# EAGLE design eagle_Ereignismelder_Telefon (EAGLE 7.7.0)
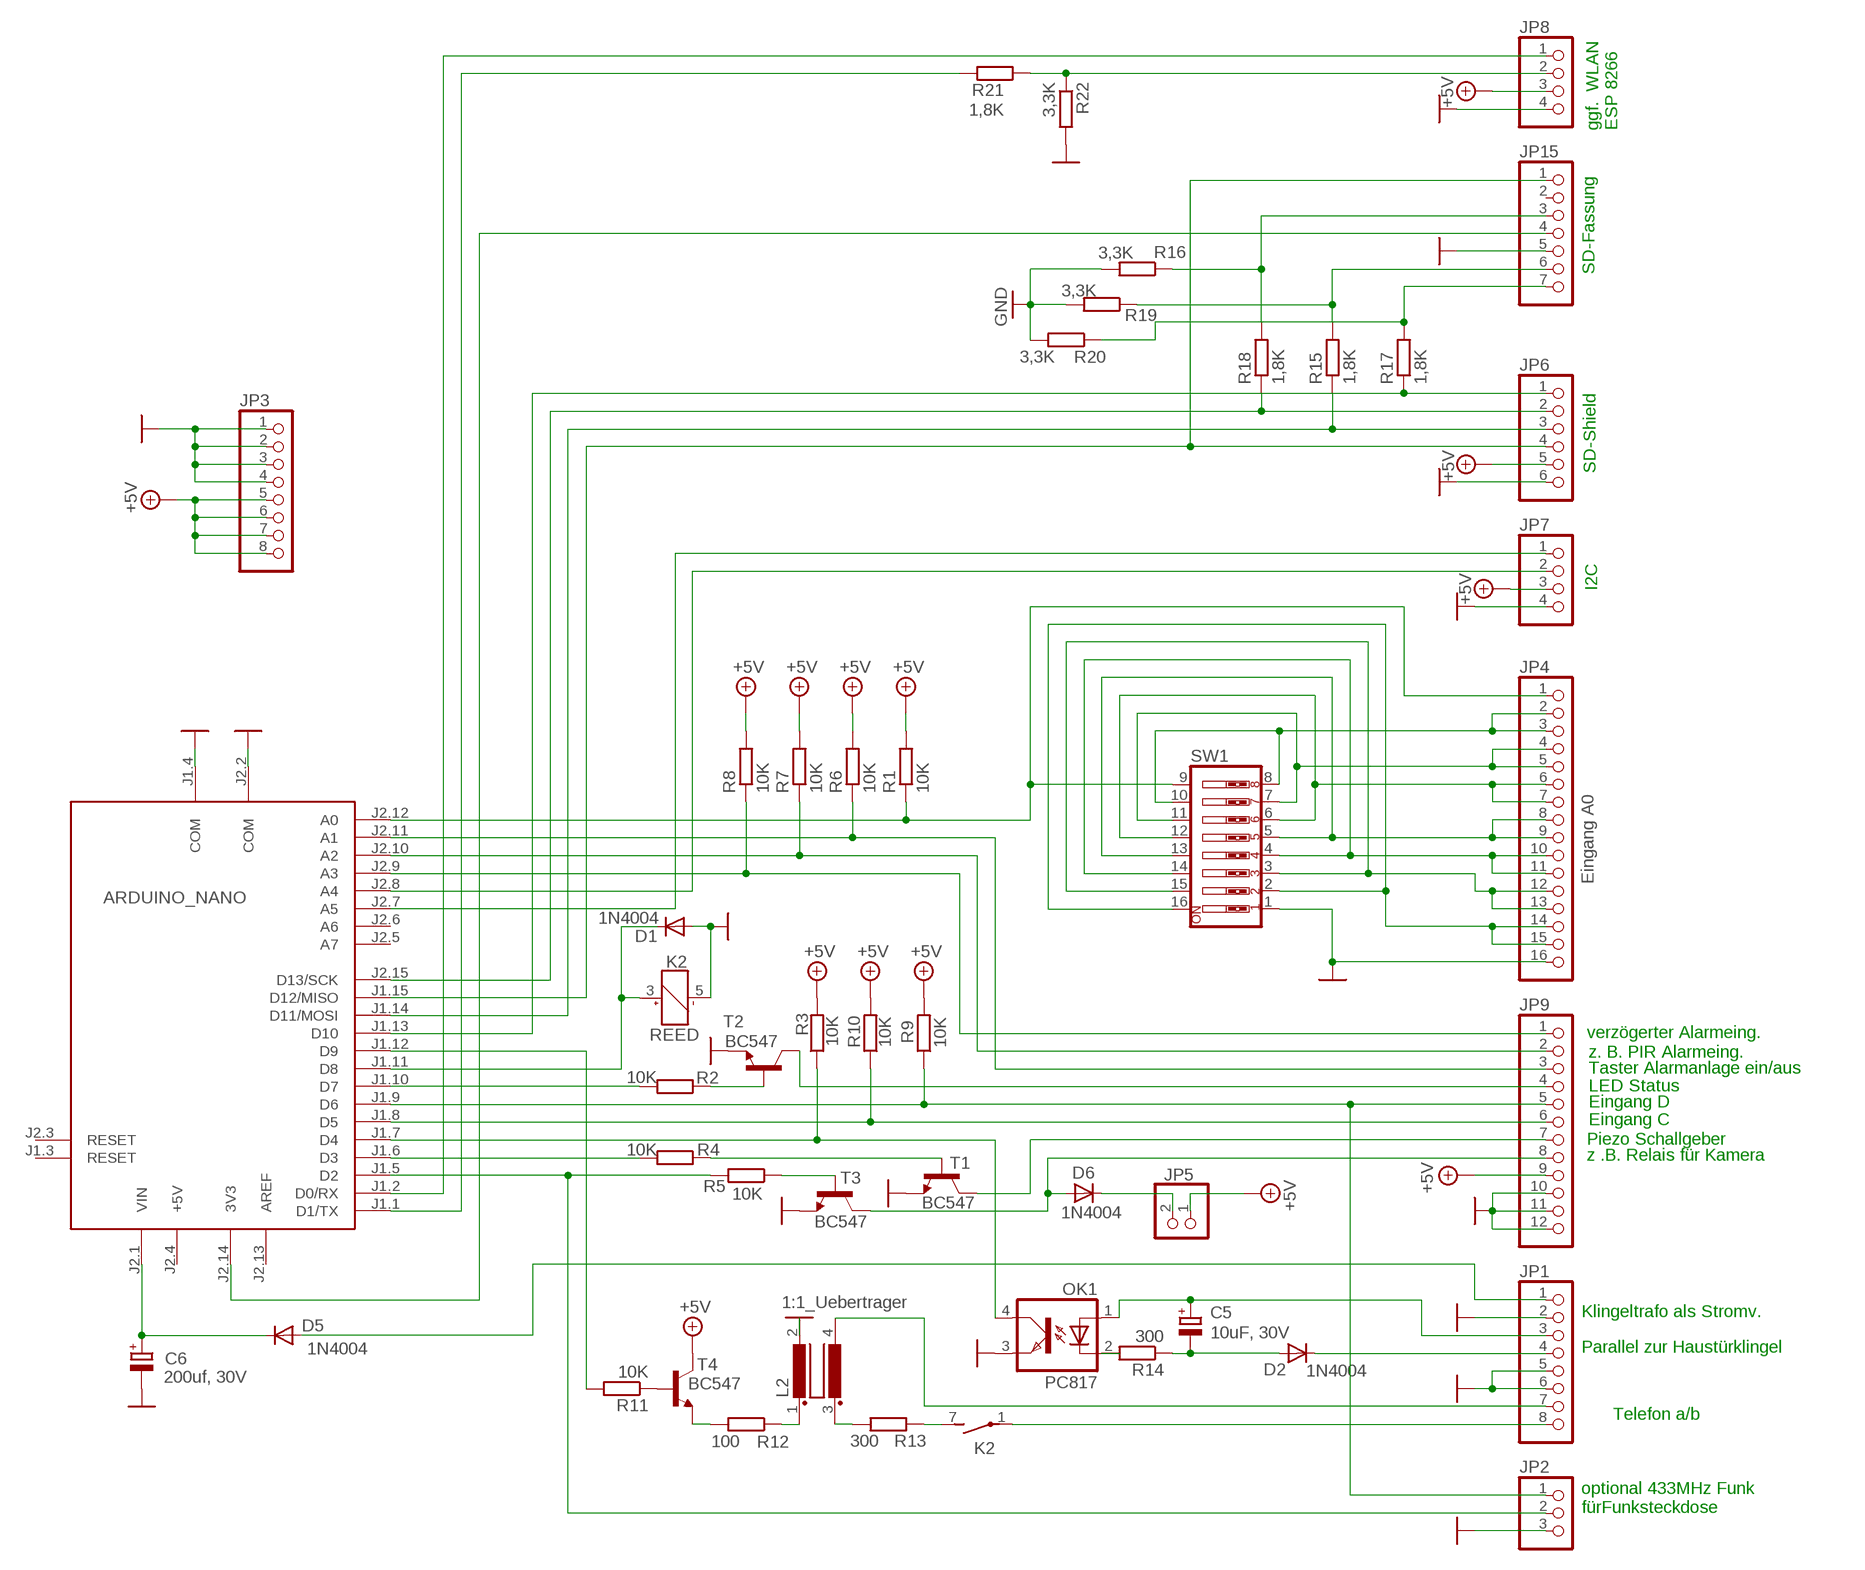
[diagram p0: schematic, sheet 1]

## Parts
C5  10uF, 30V  CPOL-EUE5-4  [E5-4]
C6  200uf, 30V  CPOL-EUE5-4  [E5-4]
D1  1N4004  [DO41-10]
D2  1N4004  [DO41-10]
D5  1N4004  [DO41-10]
D6  1N4004  [DO41-10]
JP1  PINHD-1X8  [1X08]
JP2  PINHD-1X3  [1X03]
JP3  PINHD-1X8  [1X08]
JP4  Eingang A0  PINHD-1X16  [1X16]
JP5  PINHD-1X2  [1X02]
JP6  PINHD-1X6  [1X06]
JP7  PINHD-1X4  [1X04]
JP8  PINHD-1X4  [1X04]
JP9  PINHD-1X12  [1X12]
JP15  PINHD-1X7  [1X07]
K2  REED  [REED]
L2  1:1_Uebertrager  R1405VB1/2  [B1/2]
MODUL1  ARDUINO_NANO  ARDUINO_NANO2  [ARDUINO_NANO2]
OK1  PC817  [DIL04]
R1  10K  R-EU_0204/7  [0204/7]
R2  10K  R-EU_0204/7  [0204/7]
R3  10K  R-EU_0204/7  [0204/7]
R4  10K  R-EU_0204/7  [0204/7]
R5  10K  R-EU_0204/7  [0204/7]
R6  10K  R-EU_0204/7  [0204/7]
R7  10K  R-EU_0204/7  [0204/7]
R8  10K  R-EU_0204/7  [0204/7]
R9  10K  R-EU_0204/7  [0204/7]
R10  10K  R-EU_0204/7  [0204/7]
R11  10K  R-EU_0204/7  [0204/7]
R12  100  R-EU_0204/7  [0204/7]
R13  300  R-EU_0204/7  [0204/7]
R14  300  R-EU_0204/7  [0204/7]
R15  1,8K  R-EU_0204/7  [0204/7]
R16  3,3K  R-EU_0204/7  [0204/7]
R17  1,8K  R-EU_0204/7  [0204/7]
R18  1,8K  R-EU_0204/7  [0204/7]
R19  3,3K  R-EU_0204/7  [0204/7]
R20  3,3K  R-EU_0204/7  [0204/7]
R21  1,8K  R-EU_0204/7  [0204/7]
R22  3,3K  R-EU_0204/7  [0204/7]
SW1  SW_DIP-8  [EDG-08]
T1  BC547  [TO92]
T2  BC547  [TO92]
T3  BC547  [TO92]
T4  BC547  [TO92]

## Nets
+5V: JP3.5 JP3.6 JP3.7 JP3.8 JP5.1 JP6.5 JP7.3 JP8.3 JP9.9 R1.2 R3.2 R6.2 R7.2 R8.2 R9.2 R10.2 T4.3(C)
EINGANG_A0: JP4.8 JP4.9 SW1.5 SW1.13
GND: C6.- D1.A JP1.2 JP1.5 JP1.6 JP2.3 JP3.1 JP3.2 JP3.3 JP3.4 JP4.16 JP6.6 JP7.4 JP8.4 JP9.10 JP9.11 JP9.12 JP15.5 K2.5(1:-) L2.2 MODUL1.J1.4(COM) MODUL1.J2.2(COM) OK1.3(EMIT) R16.2 R19.2 R20.2 R22.2 SW1.1 T1.1(E) T2.1(E) T3.1(E)
N$1: JP4.1 MODUL1.J2.12(A0) R1.1 SW1.9
N$2: JP8.1 MODUL1.J1.2(D0/RX)
N$3: JP4.2 JP4.3 SW1.8 SW1.10
N$4: JP9.2 MODUL1.J2.10(A2) R7.1
N$5: JP9.3 MODUL1.J2.11(A1) R6.1
N$6: JP4.6 JP4.7 SW1.6 SW1.12
N$7: JP4.10 JP4.11 SW1.4 SW1.14
N$8: JP4.12 JP4.13 SW1.3 SW1.15
N$9: MODUL1.J1.1(D1/TX) R21.2
N$10: JP9.1 MODUL1.J2.9(A3) R8.1
N$11: JP2.1 JP9.5 MODUL1.J1.9(D6) R9.1
N$12: JP9.6 MODUL1.J1.8(D5) R10.1
N$13: MODUL1.J1.7(D4) OK1.4(COL) R3.1
N$14: MODUL1.J1.6(D3) R4.2
N$15: R4.1 T1.2(B)
N$16: R5.1 T3.2(B)
N$18: JP9.7 T1.3(C)
N$19: D6.A JP9.8 T3.3(C)
N$20: D1.C K2.3(1:+) MODUL1.J1.11(D8)
N$21: R12.2 T4.1(E)
N$22: MODUL1.J1.12(D9) R11.2
N$23: R11.1 T4.2(B)
N$24: L2.1 R12.1
N$25: K2.7(2:S) R13.1
N$26: L2.3 R13.2
N$27: JP1.7 L2.4
N$28: JP1.8 K2.1(2:P)
N$29: OK1.2(C) R14.2
N$30: C5.- D2.A R14.1
N$31: D2.C JP1.4
N$32: C5.+ JP1.3 OK1.1(A)
N$33: D5.A JP1.1
N$34: C6.+ D5.C MODUL1.J2.1(VIN)
N$35: D6.C JP5.2
N$36: JP7.2 MODUL1.J2.8(A4)
N$37: JP6.4 JP15.1 MODUL1.J1.15(D12/MISO)
N$38: JP6.3 MODUL1.J1.14(D11/MOSI) R15.1
N$39: JP6.2 MODUL1.J2.15(D13/SCK) R18.1
N$40: JP6.1 MODUL1.J1.13(D10) R17.1
N$41: JP7.1 MODUL1.J2.7(A5)
N$42: JP15.6 R15.2 R19.1
N$43: JP15.7 R17.2 R20.1
N$44: JP15.3 R16.1 R18.2
N$45: JP15.4 MODUL1.J2.14(3V3)
N$46: JP4.14 JP4.15 SW1.2 SW1.16
N$47: JP4.4 JP4.5 SW1.7 SW1.11
N$48: JP8.2 R21.1 R22.1
N$49: MODUL1.J1.10(D7) R2.2
N$50: JP9.4 T2.3(C)
N$51: R2.1 T2.2(B)
N$53: JP2.2 MODUL1.J1.5(D2) R5.2
Unconnected: JP15.2 MODUL1.J1.3(RESET) MODUL1.J2.3(RESET) MODUL1.J2.5(A7) MODUL1.J2.6(A6)

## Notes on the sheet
- ggf.  WLAN
  ESP 8266
- SD-Fassung
- SD-Shield
- I2C
- verzögerter Alarmeing.
- z. B. PIR Alarmeing.
- Taster Alarmanlage ein/aus
- LED Status
- Eingang D
- Eingang C
- Piezo Schallgeber
- z .B. Relais für Kamera
- Klingeltrafo als Stromv.
- Parallel zur Haustürklingel
- Telefon a/b
- optional 433MHz Funk
  fürFunksteckdose

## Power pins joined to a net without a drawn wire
+5V: MODUL1.J2.4(+5V)
AREF: MODUL1.J2.13(AREF)

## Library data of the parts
C5 C6 = rcl:CPOL-EU: POLARIZED CAPACITOR, European symbol
D1 D2 D5 D6 = diode:1N4004: DIODE
JP1 JP3 = pinhead:PINHD-1X8: PIN HEADER
JP2 = pinhead:PINHD-1X3: PIN HEADER
JP4 = pinhead:PINHD-1X16: PIN HEADER
JP5 = pinhead:PINHD-1X2: PIN HEADER
JP6 = pinhead:PINHD-1X6: PIN HEADER
JP7 JP8 = pinhead:PINHD-1X4: PIN HEADER
JP9 = pinhead:PINHD-1X12: PIN HEADER
JP15 = pinhead:PINHD-1X7: PIN HEADER
K2 = relay:REED: RELAY reed, 1 x norm. open with polarity, grid 5.08; OC_FARNELL: unknown; OC_NEWARK: unknown
L2 = inductor-nkl:R1405V: Übertrager (verlustarm) bis typ. 400kHz Power transformer (low loss) up to typ. 400kHz; OC_FARNELL: unknown; OC_NEWARK: unknown
MODUL1 = arduino:ARDUINO_NANO2: Arduino Nano2 Auto generated by modulcreator.ulp \;; ANZAHL: 2; MODUL: TRUE; STECKX0: -76200; STECKX1: 76200; STECKY0: 177800; STECKY1: 177800
OK1 = optocoupler:PC817: SHARP OPTO COUPLER; MPN: PC817X4J000F; OC_FARNELL: 9707727; OC_NEWARK: 97K7059
R1-R22 = rcl:R-EU_: RESISTOR, European symbol
SW1 = special:SW_DIP-8: DIP SWITCH
T1-T4 = transistor:BC547: NPN TRANSISTOR

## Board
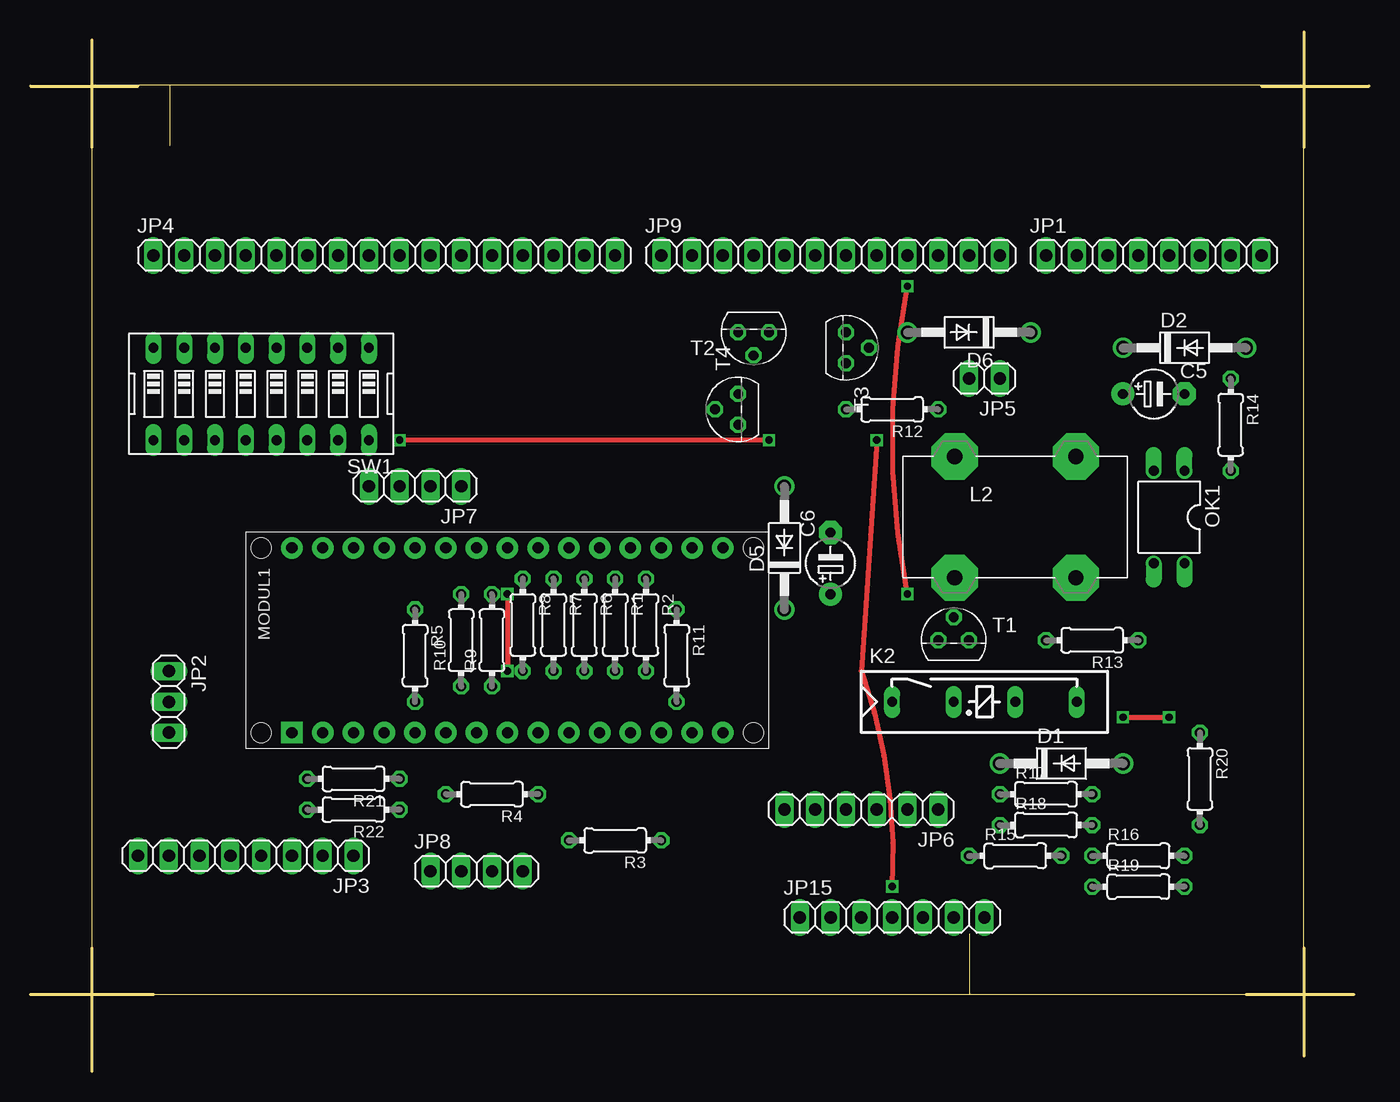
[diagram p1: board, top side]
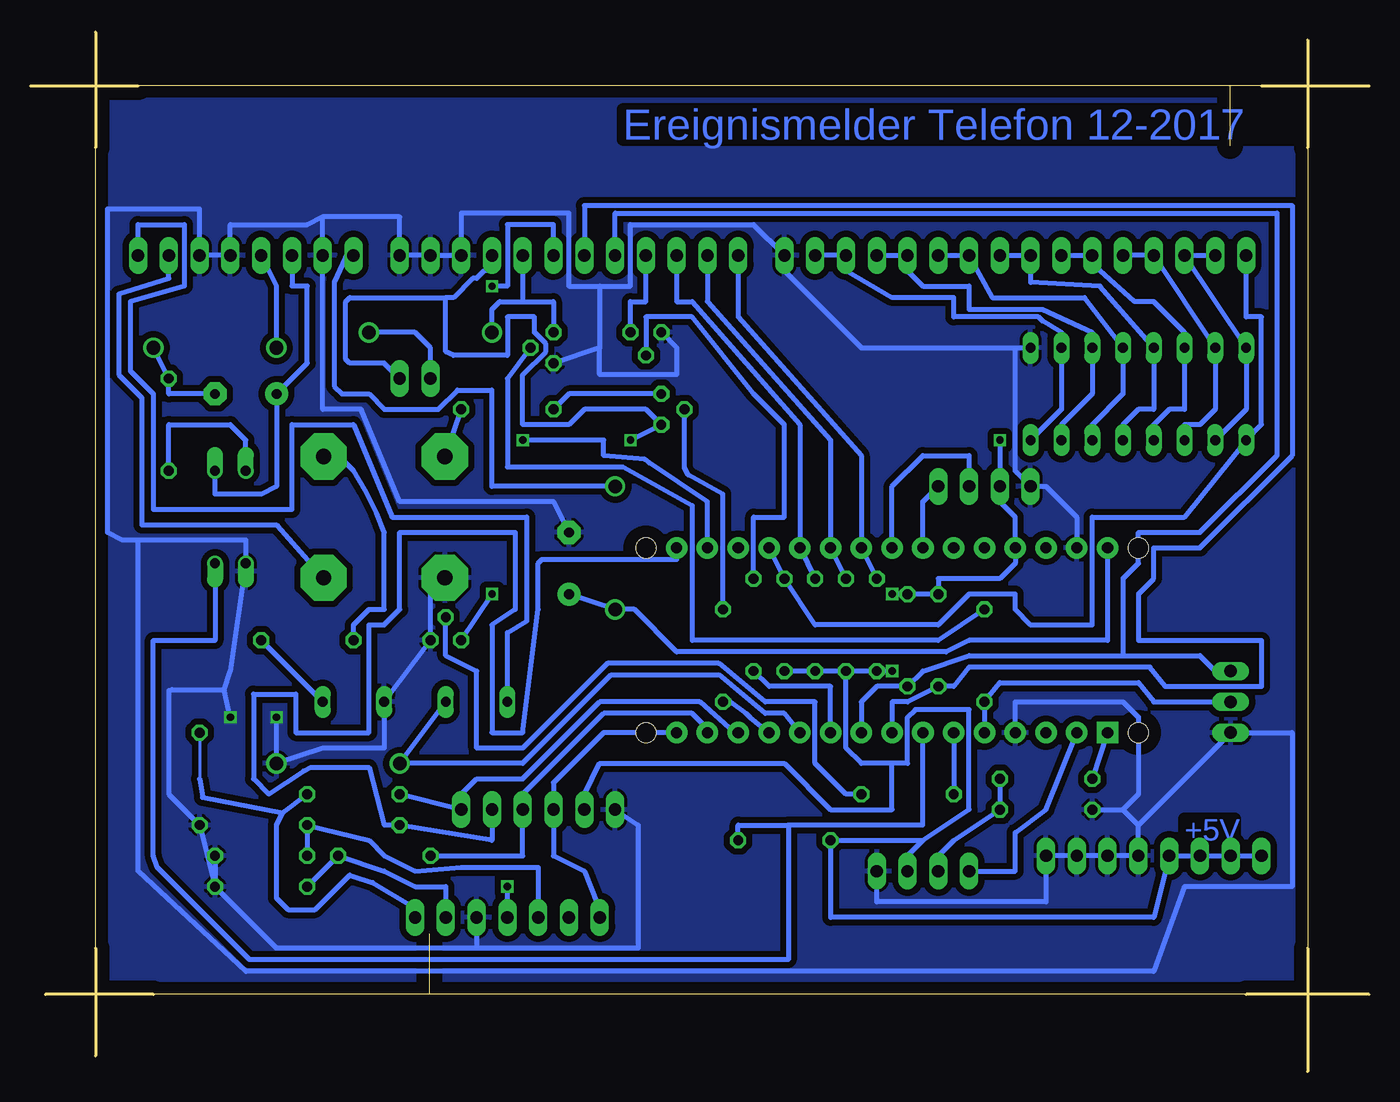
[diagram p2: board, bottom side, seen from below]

Size 110.49 x 85.72 mm. Coordinates in mm from the lower left corner, seen from the top.
Outline: 10.16,6.35 5.08,6.35 5.08,10.16
Outline: 10.16,6.35 77.54,6.35
Outline: 77.54,6.35 100.33,6.35
Outline: 100.33,6.35 105.08,6.35 105.08,81.35 11.5,81.35
Outline: 11.5,81.35 5.08,81.35 5.08,76.2
Outline: 5.08,76.2 5.08,10.16
Outline: 11.5,81.35 11.5,76.35
Outline: 77.54,6.35 77.54,11.35
Outline: 5.08,85.09 5.08,76.2
Outline: 0,81.28 8.89,81.28
Outline: 5.08,10.16 5.08,0
Outline: 0,6.35 10.16,6.35
Outline: 105.09,10.16 105.09,1.27
Outline: 100.33,6.35 109.22,6.35
Outline: 105.09,85.72 105.09,76.2
Outline: 101.6,81.28 110.49,81.28
Copper layers (1*16): Top 0.035mm / dielectric 1.5mm / Bottom 0.035mm
Design rules "default": minimum track width 10mil, minimum drill 24mil, track to track 8mil, track to pad 8mil, pad to pad 8mil, via to via 8mil, smd to smd 8mil, copper to edge 40mil, drill to drill 8mil, minimum pad ring 10mil, minimum via ring 8mil, stop-mask expansion 4mil, vias tented up to drill 0mil, thermal gap 10mil

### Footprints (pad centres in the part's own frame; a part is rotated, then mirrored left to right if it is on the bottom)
E5-4 = drill 0.813 pad 1.905: + -2.54,0 | drill 0.813 pad 1.905 octagon: - 2.54,0
DO41-10 = drill 1.118: A 5.08,0; C -5.08,0
1X08 = drill 1.016 long: 1 -8.89,0; 2 -6.35,0; 3 -3.81,0; 4 -1.27,0; 5 1.27,0; 6 3.81,0; 7 6.35,0; 8 8.89,0
1X03 = drill 1.016 long: 1 -2.54,0; 2 0,0; 3 2.54,0
1X16 = drill 1.016 long: 1 -19.05,0; 2 -16.51,0; 3 -13.97,0; 4 -11.43,0; 5 -8.89,0; 6 -6.35,0; 7 -3.81,0; 8 -1.27,0; 9 1.27,0; 10 3.81,0; 11 6.35,0; 12 8.89,0; 13 11.43,0; 14 13.97,0; 15 16.51,0; 16 19.05,0
1X02 = drill 1.016 long: 1 -1.27,0; 2 1.27,0
1X06 = drill 1.016 long: 1 -6.35,0; 2 -3.81,0; 3 -1.27,0; 4 1.27,0; 5 3.81,0; 6 6.35,0
1X04 = drill 1.016 long: 1 -3.81,0; 2 -1.27,0; 3 1.27,0; 4 3.81,0
1X12 = drill 1.016 long: 1 -13.97,0; 2 -11.43,0; 3 -8.89,0; 4 -6.35,0; 5 -3.81,0; 6 -1.27,0; 7 1.27,0; 8 3.81,0; 9 6.35,0; 10 8.89,0; 11 11.43,0; 12 13.97,0
1X07 = drill 1.016 long: 1 -7.62,0; 2 -5.08,0; 3 -2.54,0; 4 0,0; 5 2.54,0; 6 5.08,0; 7 7.62,0
REED = drill 0.813 long: 1 -17.78,2.54; 3 -12.7,2.54; 5 -7.62,2.54; 7 -2.54,2.54
B1/2 = drill 1.27 pad 3.81 octagon: 1 -5,5; 2 -5,-5; 3 5,5; 4 5,-5
ARDUINO_NANO2 = drill 0.914 pad 1.778 square: J1.1 -7.62,17.78 | drill 0.914 pad 1.778: J1.2 -7.62,15.24; J1.3 -7.62,12.7; J1.4 -7.62,10.16; J1.5 -7.62,7.62; J1.6 -7.62,5.08; J1.7 -7.62,2.54; J1.8 -7.62,0; J1.9 -7.62,-2.54; J1.10 -7.62,-5.08; J1.11 -7.62,-7.62; J1.12 -7.62,-10.16; J1.13 -7.62,-12.7; J1.14 -7.62,-15.24; J1.15 -7.62,-17.78; J2.1 7.62,17.78; J2.2 7.62,15.24; J2.3 7.62,12.7; J2.4 7.62,10.16; J2.5 7.62,7.62; J2.6 7.62,5.08; J2.7 7.62,2.54; J2.8 7.62,0; J2.9 7.62,-2.54; J2.10 7.62,-5.08; J2.11 7.62,-7.62; J2.12 7.62,-10.16; J2.13 7.62,-12.7; J2.14 7.62,-15.24; J2.15 7.62,-17.78 | hole 1.651: -7.62,-20.32; 7.62,-20.32; 7.62,20.32; -7.62,20.32
DIL04 = drill 0.813 offset: 1 -1.27,-3.81; 2 1.27,-3.81; 3 1.27,3.81; 4 -1.27,3.81
0204/7 = drill 0.813 octagon: 1 -3.81,0; 2 3.81,0
EDG-08 = drill 0.813 long: 1 -8.89,-3.81; 2 -6.35,-3.81; 3 -3.81,-3.81; 4 -1.27,-3.81; 5 1.27,-3.81; 6 3.81,-3.81; 7 6.35,-3.81; 8 8.89,-3.81; 9 8.89,3.81; 10 6.35,3.81; 11 3.81,3.81; 12 1.27,3.81; 13 -1.27,3.81; 14 -3.81,3.81; 15 -6.35,3.81; 16 -8.89,3.81
TO92 = drill 0.813 octagon: 1 1.27,0; 2 0,1.905; 3 -1.27,0

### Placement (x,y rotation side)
C5  92.71,55.88 0 top
C6  66.04,41.91 90 top
D1  85.09,25.4 0 top
D2  95.25,59.69 0 top
D5  62.23,43.18 90 top
D6  77.47,60.96 180 top
JP1  92.71,67.31 0 top
JP2  11.43,30.48 270 top
JP3  17.78,17.78 180 top
JP4  29.21,67.31 0 top
JP5  78.74,57.15 180 top
JP6  68.58,21.59 180 top
JP7  31.75,48.26 180 top
JP8  36.83,16.51 0 top
JP9  66.04,67.31 0 top
JP15  71.12,12.7 0 top
K2  88.9,27.94 0 top
L2  81.28,45.72 0 top
MODUL1  39.37,35.56 90 top
OK1  93.98,45.72 180 top
R1  48.26,36.83 270 top
R2  50.8,36.83 270 top
R3  48.26,19.05 180 top
R4  38.1,22.86 180 top
R5  31.75,34.29 270 top
R6  45.72,36.83 270 top
R7  43.18,36.83 270 top
R8  40.64,36.83 270 top
R9  38.1,35.56 90 top
R10  35.56,35.56 90 top
R11  53.34,34.29 270 top
R12  71.12,54.61 180 top
R13  87.63,35.56 180 top
R14  99.06,53.34 270 top
R15  81.28,17.78 0 top
R16  91.44,17.78 0 top
R17  83.82,22.86 0 top
R18  83.82,20.32 0 top
R19  91.44,15.24 0 top
R20  96.52,24.13 270 top
R21  26.67,24.13 180 top
R22  26.67,21.59 180 top
SW1  19.05,55.88 180 top
T1  76.2,35.56 0 top
T2  59.69,60.96 180 top
T3  67.31,59.69 270 top
T4  58.42,54.61 90 top

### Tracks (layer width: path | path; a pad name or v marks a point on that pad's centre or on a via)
+5V  (via drill 0.6)
  Top 0.406: v39.37,39.37 v39.37,33.02 | v60.96,52.07 v30.48,52.07
  Bottom 0.406: R7.2 R8.2 v39.37,33.02 | 39.37,25.4 38.1,25.4 38.1,29.21 37.46,29.84 33.02,29.84 33.02,21.59 36.83,19.05 | 39.37,25.4 41.91,25.4 43.18,26.67 R7.2 | JP6.5 64.77,22.86 63.5,25.4 48.26,25.4 44.45,21.59 39.37,21.59 39.37,25.4 | JP3.8 JP3.7 JP3.6 JP3.5 17.78,12.7 44.45,12.7 R3.2 36.83,19.05 | R7.2 R6.2 R1.2 | v39.37,39.37 R9.2 R10.2 35.56,40.64 30.48,40.64 29.21,41.91 MODUL1.J2.4 29.21,45.72 30.48,46.99 JP7.3 v30.48,52.07 | v60.96,52.07 T4.3 59.69,54.61 64.77,54.61 66.04,53.34 69.85,53.34 69.85,57.47 67.95,59.37 67.95,60.01 68.9,60.96 68.9,62.23 71.12,62.23 71.12,59.05 75.56,59.05 76.2,59.37 76.2,63.82 | 36.83,19.05 38.1,17.78 JP8.3 | JP5.1 81.28,58.42 84.14,58.42 84.45,58.74 84.45,63.5 84.14,63.82 76.2,63.82 | JP9.9 72.39,66.04 73.02,66.04 73.66,65.41 73.98,65.41 75.56,63.82 76.2,63.82
EINGANG_A0
  Bottom 0.406: SW1.13 20.32,53.34 19.05,54.61 17.78,54.61 SW1.5 22.23,64.77 27.94,65.09 JP4.8 JP4.9
GND  (via drill 0.6)
  Top 0.406: v90.17,29.21 v93.98,29.21
  Bottom 0.406: L2.2 77.47,40.8 T1.1 K2.5 81.28,26.67 86.36,26.67 D1.A v90.17,29.21 | C6.- 67.31,46.99 80.01,46.99 83.19,54.61 86.36,54.61 JP1.2 86.36,70.48 | MODUL1.J2.2 24.13,45.72 26.67,48.26 JP7.4 29.21,49.53 29.21,59.69 | MODUL1.J1.4 29.21,30.48 20.32,30.48 19.05,29.21 19.05,22.86 20.32,21.59 | R19.2 R20.2 99.06,22.86 99.06,31.43 98.81,31.5 94.49,31.5 | R19.2 90.17,10.16 73.66,10.16 | JP6.6 60.32,20.32 60.32,10.16 73.66,10.16 | 86.36,70.48 87.63,69.85 93.98,69.85 JP1.5 JP1.6 96.52,71.12 104.14,71.12 104.14,44.45 102.87,43.82 101.6,43.82 | v93.98,29.21 94.49,31.5 | 94.49,31.5 93.98,33.02 OK1.3 92.71,43.82 101.6,43.82 | 29.21,59.69 41.91,59.69 48.26,66.04 JP4.16 50.8,69.85 60.96,69.85 60.96,64.77 63.5,64.77 | 29.21,59.69 SW1.1 | T2.1 57.15,59.69 57.15,57.47 63.5,57.47 63.5,59.69 | 86.36,70.48 80.01,70.48 JP9.12 JP9.11 JP9.10 74.93,70.8 66.04,70.8 66.04,64.77 63.5,64.77 | 63.5,59.69 T3.1 | 63.5,64.77 63.5,59.69 | R16.2 R19.2 | JP8.4 40.64,13.97 26.67,13.97 JP3.1 JP3.2 JP3.3 JP3.4 19.05,20.32 | JP15.5 73.66,10.16 | 19.05,20.32 JP2.3 6.35,27.94 6.35,15.24 15.24,15.24 17.78,8.25 92.71,8.25 101.6,16.51 101.6,43.82 | R22.2 20.32,21.59 | 20.32,21.59 19.05,20.32
  pour Bottom (isolate 0.508): 5.08,81.28 105.41,81.28 105.41,6.35 5.08,6.35
N$1
  Bottom 0.406: MODUL1.J2.12 R1.1 45.72,36.83 35.56,36.83 33.02,39.37 29.21,39.37 29.21,38.1 27.94,36.83 22.86,36.83 22.86,45.72 15.24,45.72 SW1.9 8.89,53.34 8.89,62.23 10.16,62.23 JP4.1
N$2
  Bottom 0.406: MODUL1.J1.2 26.67,21.59 29.21,19.69 29.21,16.51 JP8.1
N$3
  Bottom 0.406: JP4.2 JP4.3 SW1.8 10.16,54.61 SW1.10
N$4
  Bottom 0.406: R7.1 MODUL1.J2.10 44.45,52.07 54.61,63.5 JP9.2
N$5
  Bottom 0.406: R6.1 MODUL1.J2.11 46.99,53.34 55.88,63.5 57.15,63.5 JP9.3
N$6
  Bottom 0.406: JP4.7 JP4.6 22.23,66.04 19.37,63.5 17.78,63.5 15.24,60.96 SW1.6 15.24,54.61 16.51,54.61 17.78,53.34 SW1.12
N$7
  Bottom 0.406: JP4.11 JP4.10 31.12,63.82 23.49,63.82 SW1.4 20.32,55.88 22.86,53.34 SW1.14
N$8
  Bottom 0.406: JP4.13 JP4.12 38.1,66.04 36.83,64.77 33.02,64.77 33.02,62.87 32.07,62.87 26.99,62.87 22.86,60.96 SW1.3 22.86,55.88 25.4,53.34 SW1.15
N$9
  Bottom 0.406: MODUL1.J1.1 R21.2
N$10
  Bottom 0.406: R8.1 MODUL1.J2.9 41.91,50.8 52.07,62.23 JP9.1
N$11
  Bottom 0.406: MODUL1.J1.9 41.91,30.48 40.64,31.75 R9.1 36.83,33.02 33.02,34.29 20.32,34.29 | JP9.5 62.23,70.8 7.62,70.8 7.62,50.8 13.97,44.45 19.05,44.45 19.05,41.91 20.32,40.64 20.32,34.29 | 20.32,34.29 13.97,34.29 12.7,33.02 JP2.1
N$12
  Bottom 0.406: MODUL1.J1.8 39.37,30.48 38.1,30.48 R10.1 34.29,31.75 33.02,33.34 18.1,33.34 16.83,31.75 8.89,31.75 8.89,35.56 19.05,35.56 19.05,39.37 17.78,40.64 17.78,43.18 13.97,43.18 6.35,50.8 6.35,71.44 64.77,71.44 JP9.6
N$13
  Bottom 0.406: OK1.4 95.25,35.56 100.33,35.56 100.33,17.78 100.01,16.83 92.39,9.21 47.94,9.21 47.94,20.32 | MODUL1.J1.7 36.83,20.32 47.94,20.32 | R3.1 52.07,20.32 47.94,20.32
N$14
  Bottom 0.406: MODUL1.J1.6 R4.2
N$15
  Bottom 0.406: R4.1 43.18,22.86 45.72,25.4 45.72,30.48 49.85,30.48 53.66,33.66 62.86,33.66 69.85,26.67 73.66,26.67 73.66,33.02 76.2,34.29 T1.2
N$16
  Bottom 0.406: T3.2 71.12,57.15 71.12,49.85 61.59,49.85 55.88,46.67 55.88,35.56 35.56,35.56 R5.1
N$17
  Bottom 0.152: 5.08,85.09 5.08,76.2
N$18  (via drill 0.6)
  Top 0.406: v72.39,39.37 arc-23 v72.39,64.77
  Bottom 0.406: T1.3 v72.39,39.37 | JP9.7 67.31,69.85 71.12,69.85 71.12,64.77 v72.39,64.77
N$19
  Bottom 0.406: JP9.8 69.85,63.5 | 69.85,63.5 67.31,63.5 T3.3 | D6.A 72.39,62.87 71.75,63.5 69.85,63.5
N$20
  Bottom 0.406: K2.3 D1.C 69.85,25.4 62.55,32.7 53.66,32.7 49.85,29.53 48.26,29.53 MODUL1.J1.11
N$21
  Bottom 0.406: T4.1 66.04,55.88 R12.2
N$22
  Bottom 0.406: R11.2 52.7,30.48 51.43,29.53 51.12,29.21 MODUL1.J1.12
N$23
  Bottom 0.406: R11.1 53.34,47.62 56.2,49.21 56.52,49.85 T4.2
N$24
  Bottom 0.406: R12.1 L2.1
N$25
  Bottom 0.406: K2.7 R13.1
N$26
  Bottom 0.406: R13.2 83.82,36.83 82.55,38.1 81.28,38.1 81.28,44.45 81.91,46.04 82.87,47.94 83.82,49.53 85.01,50.72 L2.3
N$27
  Bottom 0.406: L2.4 90.09,45.01 90.17,45.09 101.28,45.09 101.28,55.56 103.19,57.47 103.19,64.13 99.06,65.41 JP1.7
N$28
  Bottom 0.406: JP1.8 101.6,69.85 97.79,69.85 97.79,64.77 102.23,63.5 102.23,57.79 100.33,55.88 100.33,46.36 88.9,46.36 88.9,53.34 83.82,53.34 80.64,45.72 69.53,45.72 69.53,37.15 71.12,36.2 K2.1
N$29
  Bottom 0.406: OK1.2 92.71,52.07 93.98,53.34 99.06,53.34 R14.2
N$30
  Bottom 0.406: D2.A R14.1 99.06,55.88 C5.-
N$31
  Bottom 0.406: D2.C 90.17,64.77 JP1.4
N$32
  Bottom 0.406: OK1.1 95.25,47.62 91.44,47.62 90.17,48.26 C5.+ 87.63,58.42 87.63,64.77 88.9,64.77 JP1.3
N$33
  Bottom 0.406: JP1.1 83.82,68.58 85.41,65.09 85.41,56.52 84.77,55.88 82.55,55.88 81.28,54.61 76.83,54.61 75.25,56.2 72.39,56.2 72.39,48.26 D5.A
N$34
  Bottom 0.406: C6.+ D5.C 60.64,38.1 57.15,34.61 34.92,34.61 33.02,35.56 21.59,35.56 MODUL1.J2.1
N$35
  Bottom 0.406: JP5.2 77.47,59.69 78.74,60.96 D6.C
N$36
  Bottom 0.406: MODUL1.J2.8 39.37,48.26 36.83,50.8 33.02,50.8 JP7.2
N$37
  Bottom 0.406: MODUL1.J1.15 63.18,27.94 67.31,23.81 JP6.4 67.31,17.78 64.77,16.51 63.68,13.79 63.68,12.88 JP15.1
N$38
  Bottom 0.406: R15.1 69.85,17.78 JP6.3 69.85,22.86 63.18,29.53 55.88,29.53 54.61,28.26 MODUL1.J1.14
N$39
  Bottom 0.406: MODUL1.J2.15 57.15,42.23 68.26,42.23 68.58,41.91 68.58,38.1 69.85,27.94 72.39,27.94 72.39,36.83 70.48,38.1 70.48,44.45 80.01,44.45 80.01,38.1 81.28,36.83 82.55,36.83 82.55,27.94 88.58,27.94 88.58,31.12 92.08,31.12 92.08,24.13 90.8,22.86 87.95,24.77 87.31,25.08 82.55,25.08 81.28,20.32 R18.1 72.39,19.05 JP6.2
N$40
  Bottom 0.406: R17.1 JP6.1 74.93,22.86 73.66,24.13 69.85,24.13 63.5,30.48 55.24,30.48 52.39,27.94 MODUL1.J1.13
N$41
  Bottom 0.406: MODUL1.J2.7 36.83,46.99 JP7.1
N$42
  Bottom 0.406: R19.1 R15.2 81.28,16.51 78.74,15.24 76.2,15.24 JP15.6
N$43
  Bottom 0.254: R20.1 96.52,24.13
  Bottom 0.406: 89.66,21.34 90.17,20.32 90.17,14.29 89.22,13.34 87,13.34 84.14,16.19 82.23,15.56 79.06,13.65 79.06,13.02 JP15.7 | 89.66,21.34 R17.2 | 96.52,24.13 96.27,22.61 89.66,21.34
N$44
  Bottom 0.406: R16.1 R18.2 82.55,19.05 81.28,17.78 78.74,16.51 74.93,16.83 68.58,16.83 JP15.3
N$45  (via drill 0.6)
  Top 0.406: v69.85,52.07 68.58,33.02 arc-23 v71.12,15.24
  Bottom 0.406: MODUL1.J2.14 54.61,46.99 59.41,50.2 59.76,50.48 63.18,50.8 63.18,52.07 v69.85,52.07 | 71.18,13.91 v71.12,15.24 JP15.4
N$46
  Bottom 0.406: SW1.16 25.4,54.61 SW1.2 25.4,60.96 26.99,61.91 27.3,62.23 34.29,62.23 34.29,63.82 39.37,63.82 43.18,66.04 JP4.14 JP4.15
N$47
  Bottom 0.406: JP4.5 JP4.4 SW1.7 12.7,54.61 13.97,53.34 15.24,53.34 SW1.11
N$48
  Bottom 0.406: R21.1 R22.1 34.29,19.05 35.56,17.78 JP8.2
N$49
  Bottom 0.406: MODUL1.J1.10 44.45,31.75 49.53,31.75 R2.2
N$50
  Bottom 0.406: T2.3 60.96,63.5 59.69,63.5 JP9.4
N$51
  Bottom 0.406: T2.2 59.69,62.23 55.88,62.23 50.8,55.88 48.26,53.34 48.26,45.72 50.8,45.72 R2.1
N$52
  Bottom 0.152: 8.89,81.28 1.27,81.28
N$53
  Bottom 0.406: MODUL1.J1.5 R5.2 30.48,32.07 19.05,32.07 17.78,30.48 JP2.2
N$54
  Bottom 0.152: 109.22,81.28 101.6,81.28
N$55
  Bottom 0.152: 105.09,76.2 105.09,85.72
N$56
  Bottom 0.152: 105.09,10.16 105.09,2.54
N$57
  Bottom 0.152: 101.6,6.35 109.22,6.35
N$58
  Bottom 0.152: 8.89,6.35 1.27,6.35
N$59
  Bottom 0.152: 5.08,10.16 5.08,2.54

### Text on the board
Bottom: Ereignismelder Telefon 12-2017 | +5V | +5V | +5V
tValues: 1 | 5 | 9 | ~~ | bell | GND | a/b | 1 | 5 | 9 | 1 / 2 | 1 / 3 | 1 / 6 | Ereignismelder / Telefon 12-2017 / (Alarmanlage / / Haustürklingel) | 1 | I2C | USB | 433MHz | GND | +5V | GND | SD-Shield | GND | SD-Fassung | GND | ESP8266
